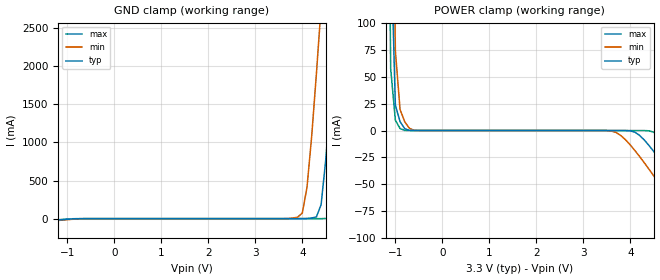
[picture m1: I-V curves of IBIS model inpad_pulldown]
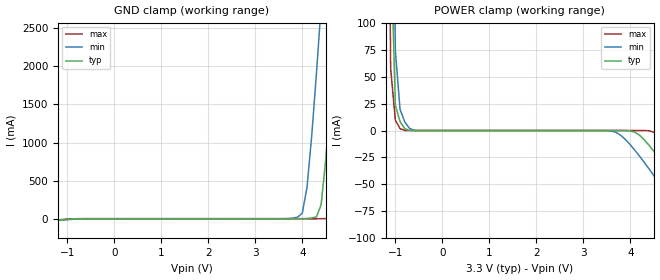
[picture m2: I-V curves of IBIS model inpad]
[IBIS Ver]   2.1
[File Name]   dac904e.ibs
[File Rev]   1.1
[Source]   Preliminary IBIS Model Generated Manually
[Notes]
   Package information estimated
[Disclaimer]   This information is for modeling purposes only
[Copyright]   (c) 2004, Texas Instruments Inc.
[Component]   tssop28
[Manufacturer]   Texas Instruments
[Package]
| Variable   Typ   Min   Max
R_pkg   0.1   0.1   0.1
L_pkg   3.0nH   3.0nH   3.0nH
C_pkg   3.0pF   3.0pF   3.0pF
[Pin]   signal_name   model_name   R_pin  L_pin   C_pin
   1   bit1   inpad   0.1   3.0nH   3.0pF
   2   bit2   inpad   0.1   3.0nH   3.0pF
   3   bit3   inpad   0.1   3.0nH   3.0pF
   4   bit4   inpad   0.1   3.0nH   3.0pF
   5   bit5   inpad   0.1   3.0nH   3.0pF
   6   bit6   inpad   0.1   3.0nH   3.0pF
   7   bit7   inpad   0.1   3.0nH   3.0pF
   8   bit8   inpad   0.1   3.0nH   3.0pF
   9   bit9   inpad   0.1   3.0nH   3.0pF
   10   bit10   inpad   0.1   3.0nH   3.0pF
   11   bit11   inpad   0.1   3.0nH   3.0pF
   12   bit12   inpad   0.1   3.0nH   3.0pF
|  13   bit13   inpad   0.1   3.0nH   3.0pF
|  14   bit14   inpad   0.1   3.0nH   3.0pF
   15   pd   inpad_pulldown   0.1   3.0nH   3.0pF
   16   int_ext_n   inpad   0.1   3.0nH   3.0pF
|  17   refin   0.1   3.0nH   3.0pF
|  18   fsa   0.1   3.0nH   3.0pF
|  19   bw   0.1   3.0nH   3.0pF
   20   agnd   GND   0.1   3.0nH   3.0pF
|  21   ioutb   0.1   3.0nH   3.0pF
|  22   iout   0.1   3.0nH   3.0pF
|  23   byp   0.1   3.0nH   3.0pF
   24   va   POWER   0.1   3.0nH   3.0pF
|  25   nc   0.1   3.0nH   3.0pF
   26   dgnd   GND   0.1   3.0nH   3.0pF
   27   vd   POWER   0.1   3.0nH   3.0pF
   28   clk   inpad   0.1   3.0nH   3.0pF
| End of package information
| Models and submodels in the file (2): inpad_pulldown (Input), inpad (Input)
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|   Model inpad_pulldown
[Model]   inpad_pulldown
Model_type   Input
Polarity   Non-Inverting
| signals   A, Y
Vinl = 0.8V
Vinh = 2.4V
|   typ   min   max
C_comp   1.5p   1.5p   1.5p
|   typ   min   max
[Temperature Range]   25   -40.0   100
|   typ   min   max
[Voltage Range]   3.30V   3.00V   3.60V
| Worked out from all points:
|   GND clamp passes 1 mA (typ) near -0.75 V on its own axis
|   POWER clamp passes 1 mA (typ) near -0.76 V on its own axis
[GND_clamp]
|   Voltage   I(typ)   I(min)   I(max)
-3.3V     -158.5mA   -161.4mA   -157.9mA
3.9V      30.05uA    19.39mA    61.51uA
4V        103.4uA    74.36mA    61.52uA
4.1V      1.676mA    412.8mA    61.53uA
4.3V      23.36mA    1.904A     61.78uA
4.4V      183.2mA    2.781A     93.91uA
4.6V      1.593A     4.618A     9.616mA
4.7V      2.478A     5.558A     57.23mA
4.8V      3.396A     6.507A     539.3mA
5V        5.282A     8.424A     2.248A
5.1V      6.239A     9.389A     3.178A
6.6V      20.93A     24.09A     17.83A
[POWER_clamp]
|   Voltage   I(typ)   I(min)   I(max)
-3.3V     20.93A     21.13A     20.8A
-1.2V     781.3mA    1.091A     542.4mA
-1.1V     183.1mA    415.5mA    57.79mA
-1V       23.53mA    74.33mA    9.622mA
-900mV    8.243mA    19.54mA    1.841mA
-800mV    1.684mA    8.075mA    95.56uA
3.6V      -8.63uA    -505.8uA   -17.55nA
4.5V      -19.53mA   -42.23mA   -1.612mA
5.3V      -70.09mA   -93.97mA   -47.16mA
5.7V      -96.89mA   -120.7mA   -74.17mA
6V        -117.3mA   -141mA     -94.83mA
6.6V      -158.5mA   -182mA     -136.7mA
|   Model inpad
[Model]   inpad
Model_type   Input
Polarity   Non-Inverting
| signals   A, Y
Vinl = 0.8V
Vinh = 2.4V
|   typ   min   max
C_comp   1.5p   1.5p   1.5p
|   typ   min   max
[Temperature Range]   25   -40.0   100
|   typ   min   max
[Voltage Range]   3.30V   3.00V   3.60V
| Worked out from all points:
|   GND clamp passes 1 mA (typ) near -0.76 V on its own axis
|   POWER clamp passes 1 mA (typ) near -0.76 V on its own axis
[GND_clamp]
|   Voltage   I(typ)   I(min)   I(max)
-3.3V     -157.3mA   -160.6mA   -155.8mA
3.9V      1.86uA     19.39mA    1.049nA
4V        79.71uA    74.36mA    1.103nA
4.1V      1.665mA    412.8mA    1.203nA
4.3V      23.35mA    1.904A     272.1nA
4.4V      183.1mA    2.781A     36.47uA
4.6V      1.593A     4.618A     9.6mA
4.7V      2.478A     5.558A     57.21mA
4.8V      3.396A     6.507A     539.2mA
5V        5.282A     8.424A     2.248A
5.1V      6.239A     9.389A     3.178A
6.6V      20.93A     24.09A     17.83A
[POWER_clamp]
|   Voltage   I(typ)   I(min)   I(max)
-3.3V     20.93A     21.13A     20.8A
-1.2V     781.3mA    1.091A     542.4mA
-1.1V     183.1mA    415.5mA    57.77mA
-1V       23.53mA    74.33mA    9.607mA
-900mV    8.236mA    19.54mA    1.814mA
-800mV    1.673mA    8.072mA    38.26uA
3.6V      -2.496nA   -470.2uA   -1.105nA
4.5V      -19.26mA   -41.88mA   -1.534mA
5.3V      -69.48mA   -93.39mA   -46.4mA
5.7V      -96.11mA   -120mA     -73.08mA
6.1V      -123.1mA   -147mA     -100.4mA
6.6V      -157.3mA   -181mA     -134.9mA
